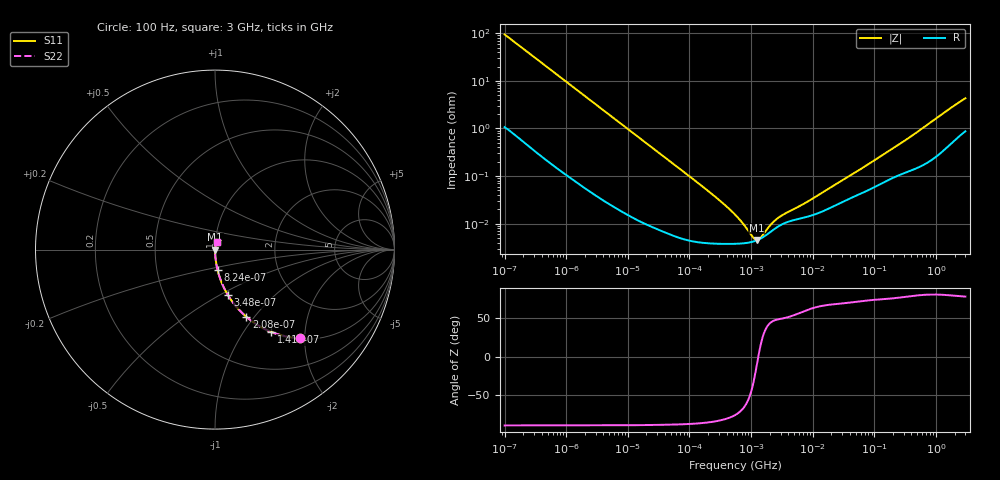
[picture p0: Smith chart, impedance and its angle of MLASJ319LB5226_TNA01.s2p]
! MLASJ319LB5226_TNA01  S-PARAMETER MODEL  ( Standard Model )
! Model Generated by TAIYO YUDEN Corporation (http://www.ty-top.com)
! Version 1.0
! TAIYO YUDEN Control No. 220601
! Copyright(c) 2009 TAIYO YUDEN CO.,LTD. All Rights Reserved.
! Product Description (link to TY-COMPAS)
! https://ds.yuden.co.jp/TYCOMPAS/or/detail?pn=MLASJ319LB5226MTNA01&u=M
! Products Name : Multilayer Ceramic Capacitors
! Characteristics :
!  Capacitance : 22 [uF] , Rated Voltage : 6.3 [V] , TCC : X5R
!  Case Size : 3.2 x 1.6 / 0.126 x 0.063 [mm/inch] , Thickness : 0.85 / 0.033 [mm/inch]
!  (Conditions: Temperature = 25 [degC] , DC Bias Voltage = 0 [V])
! External Node Assignments :
!  1  o---| |---o  2
! GND o---------o GND
! Frequency Range : 100Hz  -  3GHz  [ 401 STEP ]
# MHZ S RI R 50
! Freq[MHz].  S11 Real  S11 Imag  S21 Real  S21 Imag  S12 Real  S12 Imag  S22 Real  S22 Imag
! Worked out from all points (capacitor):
!   401 points, 100 Hz to 3 GHz, reference 50 ohm
!   read as one part in series: C = 16.8 uF near 109 Hz
!   lowest |Z| = 4.54 mohm at 1.241 MHz (marker M1)
!   series resonance near 1.307 MHz, so ESL is about 880 pH
!   S11 on the Smith chart (normalised r, x): 100 Hz: 1.02, -1.89; 141 Hz: 1.02, -1.34; 208 Hz: 1.01, -0.91; 348 Hz: 1.01, -0.55; 824 Hz: 1.00, -0.23; 3 GHz: 1.02, +0.08
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0.0001  0.4716 -0.4936  0.5284 0.4936  0.5284 0.4936  0.4716 -0.4936
0.000141  0.3125 -0.4579  0.6875 0.4579  0.6875 0.4579  0.3125 -0.4579
0.000208  0.1755 -0.3749  0.8245 0.3749  0.8245 0.3749  0.1755 -0.3749
0.000348  0.072 -0.2531  0.928 0.2531  0.928 0.2531  0.072 -0.2531
0.000824  0.0146 -0.1145  0.9854 0.1145  0.9854 0.1145  0.0146 -0.1145
0.001788  0.0035 -0.0536  0.9965 0.0536  0.9965 0.0536  0.0035 -0.0536
0.005476  0.000553 -0.0177  0.9994 0.0177  0.9994 0.0177  0.000553 -0.0177
0.031977  8.33e-05 -0.00308  0.9999 0.00308  0.9999 0.00308  8.33e-05 -0.00308
0.231582  3.84e-05 -0.000417  1 0.000417  1 0.000417  3.84e-05 -0.000417
0.388167  3.76e-05 -0.000235  1 0.000235  1 0.000235  3.76e-05 -0.000235
0.547723  3.78e-05 -0.000151  1 0.000151  1 0.000151  3.78e-05 -0.000151
0.679242  3.83e-05 -0.000108  1 0.000108  1 0.000108  3.83e-05 -0.000108
0.772864  3.88e-05 -8.47e-05  1 8.47e-05  1 8.47e-05  3.88e-05 -8.47e-05
1.240863  4.47e-05 -7.97e-06  1 7.97e-06  1 7.97e-06  4.47e-05 -7.97e-06
1.992254  6.49e-05 6.12e-05  0.9999 -6.12e-05  0.9999 -6.12e-05  6.49e-05 6.12e-05
2.171352  7.06e-05 7.23e-05  0.9999 -7.23e-05  0.9999 -7.23e-05  7.06e-05 7.23e-05
3.339322  0.0001 0.00012  0.9999 -0.00012  0.9999 -0.00012  0.0001 0.00012
9.794414  0.00015 0.000296  0.9998 -0.000296  0.9998 -0.000296  0.00015 0.000296
175.1444  0.000856 0.00331  0.9991 -0.00331  0.9991 -0.00331  0.000856 0.00331
414.2403  0.00139 0.00701  0.9986 -0.00701  0.9986 -0.00701  0.00139 0.00701
1868.531  0.00592 0.0281  0.9941 -0.0281  0.9941 -0.0281  0.00592 0.0281
3000  0.0104 0.0416  0.9896 -0.0416  0.9896 -0.0416  0.0104 0.0416
